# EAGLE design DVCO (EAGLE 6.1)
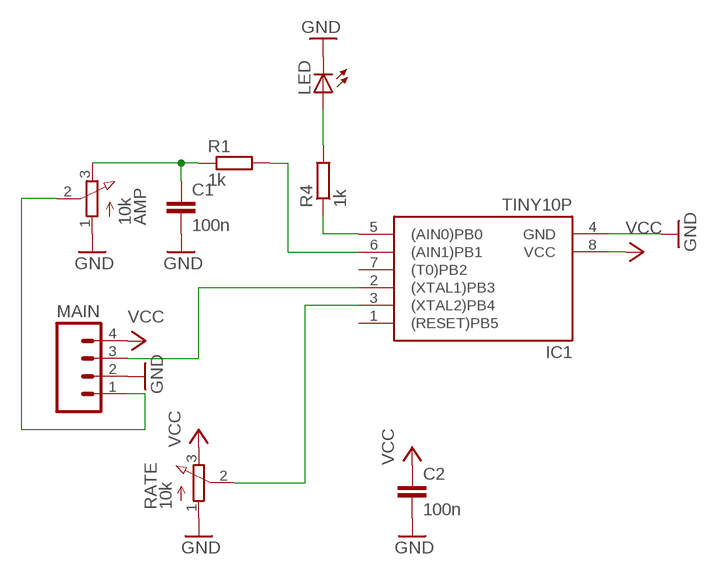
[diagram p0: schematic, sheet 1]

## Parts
AMP  10k  3RP/1610N  [3RP/1610N]
C1  100n  C-EU050-025X075  [C050-025X075]
C2  100n  C-EU050-025X075  [C050-025X075]
IC1  TINY10P  [DIL08]
LED  LED3MM  [LED3MM]
MAIN  M04  [04P]
R1  1k  R-EU_0207/10  [0207/10]
R4  1k  R-EU_0207/10  [0207/10]
RATE  10k  3RP/1610N  [3RP/1610N]

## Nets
GND: AMP.1(A) C1.2 C2.2 IC1.4(GND) LED.K(C) MAIN.2 RATE.1(A)
N$1: IC1.2((XTAL1)PB3) MAIN.3
N$2: IC1.6((AIN1)PB1) R1.2
N$3: AMP.2(S) MAIN.1
N$4: AMP.3(E) C1.1 R1.1
N$5: IC1.3((XTAL2)PB4) RATE.2(S)
N$6: IC1.5((AIN0)PB0) R4.1
N$7: LED.A R4.2
VCC: C2.1 IC1.8(VCC) MAIN.4 RATE.3(E)
Unconnected: IC1.1((RESET)PB5) IC1.7((T0)PB2)

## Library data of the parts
AMP RATE = pot:3RP/1610N: 16mm Potentiometer one level Source: http://www.alphapotentiometers.net/html/16mm_pot_2.html
C1 C2 = rcl:C-EU: CAPACITOR, European symbol
IC1 = atmel:TINY10: MICROCONTROLLER 1 Kbytes ROM; OC_FARNELL: unknown; OC_NEWARK: unknown
LED = adafruit:LED: LED
MAIN = con-amp-quick:M04: AMP QUICK CONNECTOR; OC_FARNELL: unknown; OC_NEWARK: unknown
R1 R4 = rcl:R-EU_: RESISTOR, European symbol

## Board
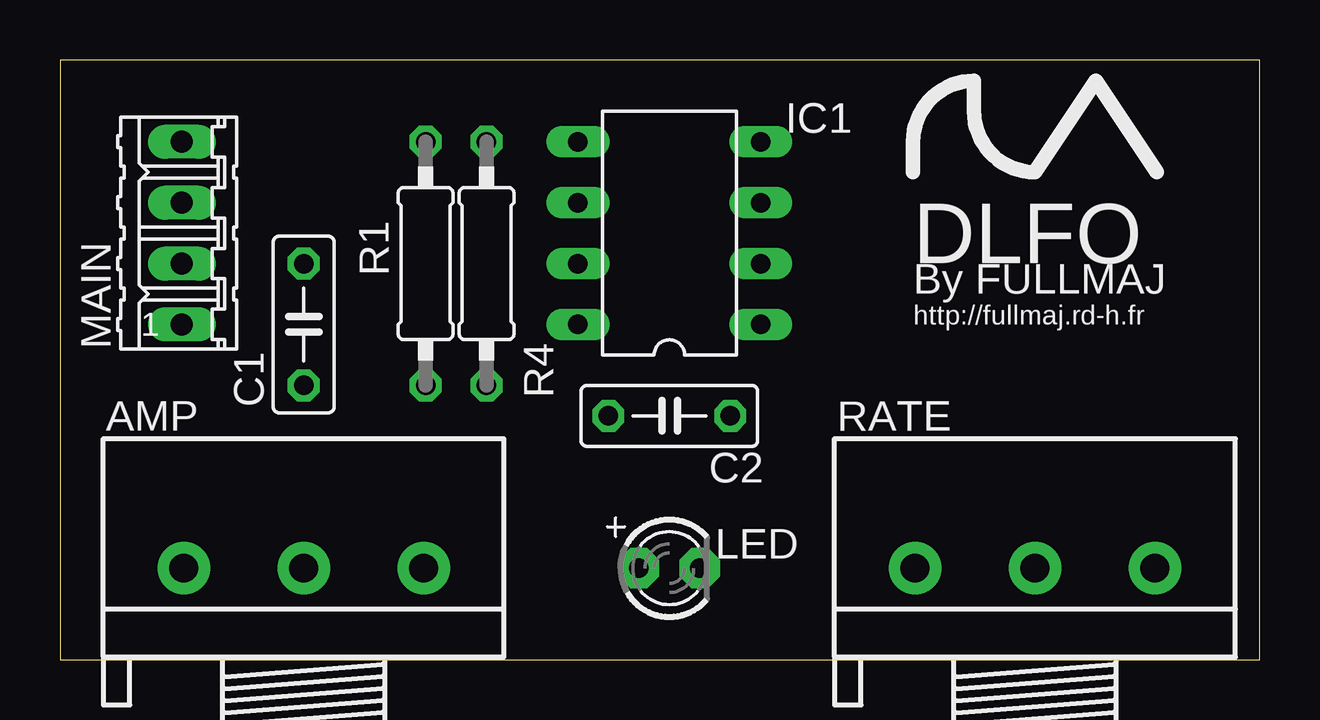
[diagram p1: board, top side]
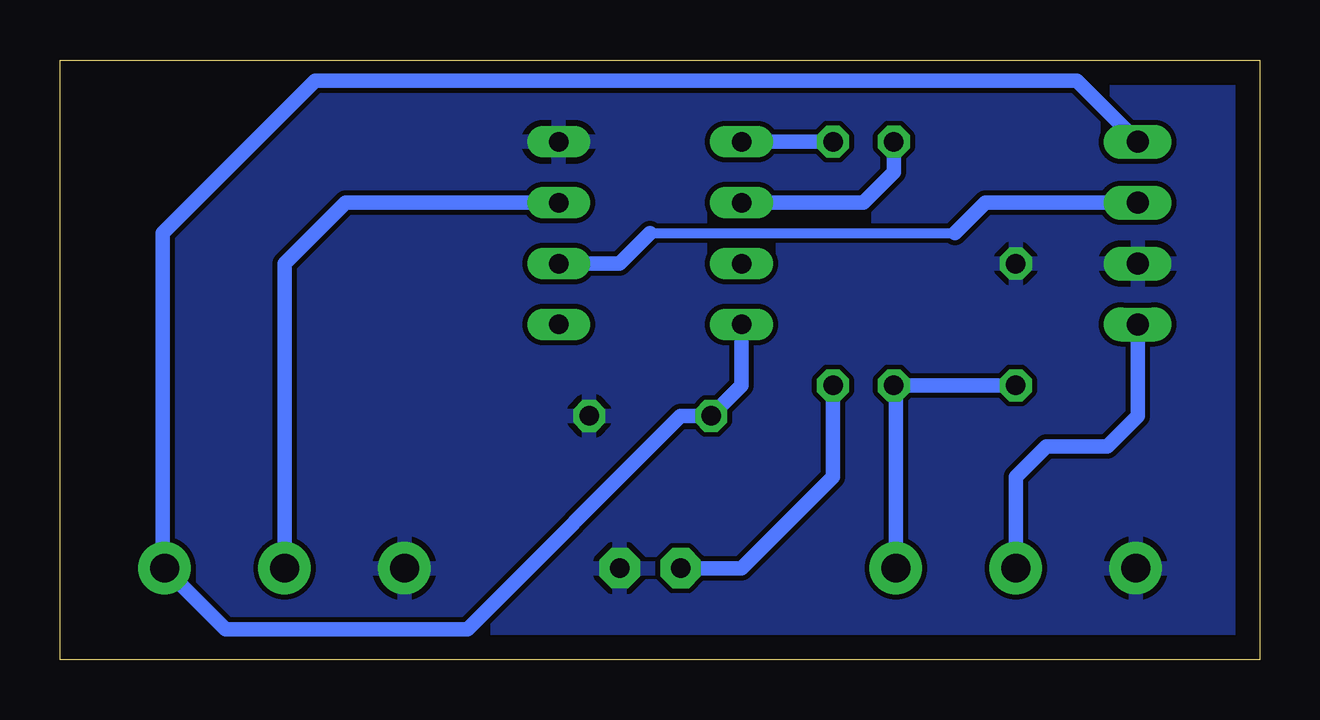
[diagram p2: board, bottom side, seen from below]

Size 50 x 25 mm. Coordinates in mm from the lower left corner, seen from the top.
Outline: 0,0 50,0 50,25 0,25 0,0
Copper layers (1*16): Top 0.035mm / dielectric 1.5mm / Bottom 0.035mm
Design rules: minimum track width 10mil, minimum drill 24mil, track to track 8mil, track to pad 8mil, pad to pad 8mil, via to via 8mil, smd to smd 8mil, copper to edge 40mil, drill to drill 8mil, minimum pad ring 10mil, minimum via ring 8mil, stop-mask expansion 4mil, vias tented up to drill 0mil, thermal gap 10mil

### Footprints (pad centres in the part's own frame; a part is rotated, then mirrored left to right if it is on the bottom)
3RP/1610N = drill 1.2 pad 2.184: 1 -5,0; 2 0,0; 3 5,0
C050-025X075 = drill 0.813 octagon: 1 -2.54,0; 2 2.54,0
DIL08 = drill 0.813 long: 1 -3.81,-3.81; 2 -1.27,-3.81; 3 1.27,-3.81; 4 3.81,-3.81; 5 3.81,3.81; 6 1.27,3.81; 7 -1.27,3.81; 8 -3.81,3.81
LED3MM = drill 0.813 pad 1.676 octagon: A -1.27,0; K 1.27,0
04P = drill 0.914 long: 1 -3.81,0; 2 -1.27,0; 3 1.27,0; 4 3.81,0
0207/10 = drill 0.813 octagon: 1 -5.08,0; 2 5.08,0

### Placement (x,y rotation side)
AMP  10.16,3.81 0 top
C1  10.16,13.97 90 top
C2  25.4,10.16 0 top
IC1  25.4,17.78 90 top
LED  25.4,3.81 0 top
MAIN  5.08,17.78 90 top
R1  15.24,16.51 90 top
R4  17.78,16.51 270 top
RATE  40.64,3.81 0 top

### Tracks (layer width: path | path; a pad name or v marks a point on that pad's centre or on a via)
GND
  pour Bottom: 0,24.13 0,0 49.53,0 49.53,24.13
N$1
  Bottom 0.406: 25.4,17.78 12.7,17.78
  Bottom 0.61: IC1.2 26.67,16.51 25.4,17.78 | 12.7,17.78 11.43,19.05 MAIN.3
N$2
  Bottom 0.61: R1.2 15.24,20.32 16.51,19.05 IC1.6
N$3
  Bottom 0.61: MAIN.1 5.08,10.16 6.35,8.89 8.89,8.89 10.16,7.62 AMP.2
N$4
  Bottom 0.61: AMP.3 15.16,11.35 R1.1 C1.1
N$5
  Bottom 0.61: IC1.3 38.1,19.05 40.64,16.51 RATE.2
N$6
  Bottom 0.61: R4.1 IC1.5
N$7
  Bottom 0.61: LED.A 21.59,3.81 17.78,7.62 R4.2
VCC
  Bottom 0.61: MAIN.4 7.62,24.13 39.37,24.13 45.72,17.78 45.72,3.89 RATE.3 43.1,1.27 33.02,1.27 24.13,10.16 C2.1 21.59,11.43 IC1.8

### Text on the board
tPlace: DLFO | By FULLMAJ | http://fullmaj.rd-h.fr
